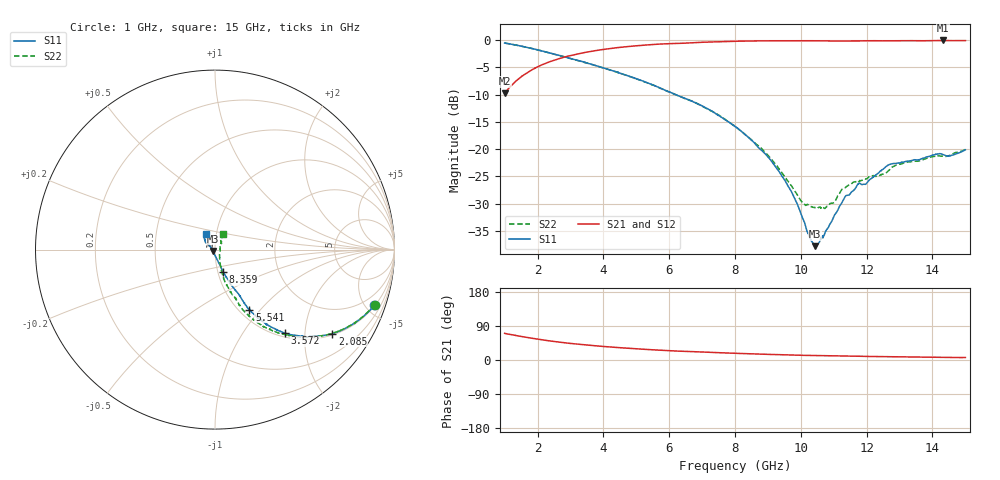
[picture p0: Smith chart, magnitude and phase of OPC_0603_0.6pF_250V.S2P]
! FILE NAME
! DATE 08/21/2012  14:57
! CORRECTED  DATA
# GHz  S  MA  R  50.00
!  FREQ  S11M  S11A  S21M  S21A  S12M  S12A  S22M  S22A
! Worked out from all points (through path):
!   1601 points, 1 GHz to 15 GHz, reference 50 ohm
!   highest |S21| = -0.05 dB at 14.33 GHz (marker M1); lowest = -9.7 dB at 1 GHz (marker M2)
!   lowest |S11| = -37.8 dB at 10.42 GHz (marker M3), VSWR 1.03, Z = 48.9 - j0.674 ohm
!   |S11| at or under -10 dB: 6.201 GHz to end of sweep
!   |S22| runs from -30.9 to -0.5 dB; largest |S21 - S12| = 0.0082
!   S11 on the Smith chart (normalised r, x): 1 GHz: 1.06, -5.73; 2.085 GHz: 1.04, -2.76; 3.572 GHz: 1.07, -1.59; 5.541 GHz: 1.11, -0.87; 8.359 GHz: 1.06, -0.27; 15 GHz: 0.89, +0.15
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1  0.9409 -19.2  0.3267 70.3  0.3265 70.3  0.9409 -19.0
1.51625  0.8798 -27.6  0.4638 61.9  0.4631 61.9  0.8797 -27.5
2.085  0.8035 -35.6  0.5851 53.9  0.5846 54.0  0.8035 -35.5
3.33625  0.6384 -48.0  0.7597 40.9  0.7591 40.9  0.6364 -48.9
3.5725  0.6082 -49.9  0.7839 39.0  0.7832 39.0  0.6073 -50.9
5.54125  0.3849 -60.3  0.9138 26.7  0.9134 26.7  0.3829 -64.5
5.6725  0.3698 -60.8  0.9191 26.1  0.9191 26.1  0.3685 -65.4
7.0375  0.2462 -63.9  0.9573 20.9  0.9572 21.0  0.2448 -70.2
8  0.1613 -67.7  0.9776 17.7  0.9763 17.8  0.1618 -73.5
8.35875  0.1323 -69.6  0.9803 16.7  0.9798 16.7  0.1324 -73.1
9.00625  0.08454 -73.2  0.9866 14.9  0.9855 14.9  0.08733 -70.2
9.51375  0.05178 -79.5  0.9889 13.7  0.9886 13.7  0.05579 -62.5
10.0475  0.0236 -100.4  0.9885 12.4  0.9881 12.4  0.03246 -36.4
10.33625  0.0141 -133.2  0.9878 11.8  0.9871 11.8  0.02964 -14.5
10.42375  0.01287 -147.7  0.987 11.6  0.9866 11.6  0.02911 -8.3
10.56375  0.01407 -172.6  0.9862 11.3  0.9858 11.3  0.02947 1.7
10.98375  0.02342 154.0  0.9824 10.6  0.9816 10.6  0.03204 29.6
11.36  0.03712 144.6  0.9828 10.3  0.9825 10.3  0.04454 41.9
12.6725  0.07181 139.9  0.9864 8.5  0.9855 8.6  0.06361 61.2
13.18875  0.07714 135.6  0.9885 7.9  0.9883 7.9  0.07528 59.7
14.32625  0.08912 126.2  0.9939 6.7  0.9931 6.7  0.08613 59.9
15  0.09866 120.4  0.9914 6.6  0.9908 6.6  0.0994 64.2
